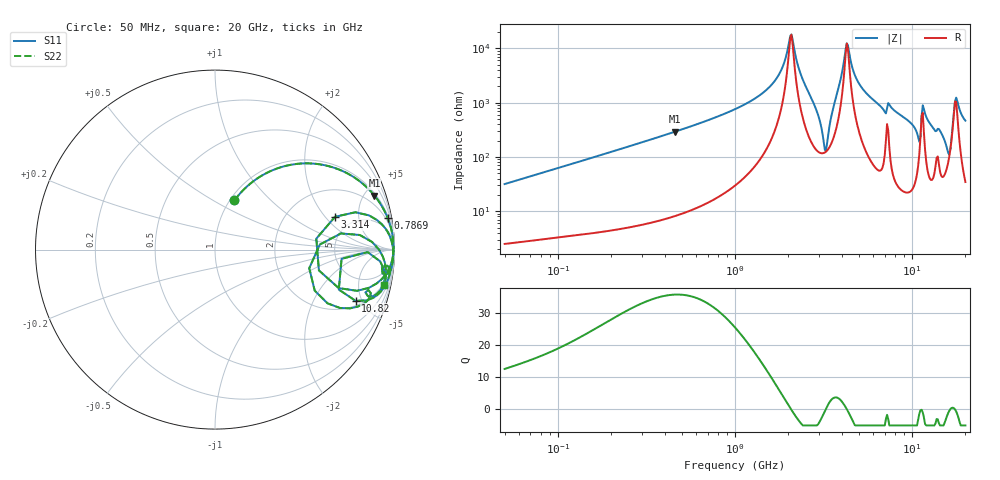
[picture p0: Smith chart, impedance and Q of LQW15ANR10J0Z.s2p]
!Murata Part Number: LQW15ANR10J0Z
!These Parameters are Measured in Series Mode Connection
!  o--[Z]--o
!Port1  Port2
!  o-------o
!Freq. Start=50[MHz] Stop=20[GHz], 401[Steps]
# Hz S RI R 50
!Freq.(Hz) S11(Real) S11(Imag) S21(Real) S21(Imag) S12(Real) S12(Imag) S22(Real) S22(Imag)
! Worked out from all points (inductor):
!   401 points, 50 MHz to 20 GHz, reference 50 ohm
!   read as one part in series: L = 99.7 nH near 51.52 MHz
!   highest Q = 35.8 at 458.9 MHz (marker M1), where L = 101 nH
!   self-resonance near 2.052 GHz
!   S11 on the Smith chart (normalised r, x): 50 MHz: 1.05, +0.63; 786.9 MHz: 1, +11; 3.314 GHz: 3.63, +2.56; 10.82 GHz: 2.37, -4.45; 20 GHz: 1.69, -9.30
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5e7  0.1085 0.274  0.8915 -0.274  0.8915 -0.274  0.1085 0.274
1.364002e8  0.4206 0.4722  0.5794 -0.4722  0.5794 -0.4722  0.4206 0.4722
3.721004e8  0.8382 0.3542  0.1618 -0.3542  0.1618 -0.3542  0.8382 0.3542
4.589149e8  0.8884 0.3013  0.1116 -0.3013  0.1116 -0.3013  0.8884 0.3013
7.868965e8  0.9621 0.1755  0.0379 -0.1755  0.0379 -0.1755  0.9621 0.1755
1e9  0.978 0.1283  0.022 -0.1283  0.022 -0.1283  0.978 0.1283
1.639343e9  0.9934 0.0429  0.00658 -0.0429  0.00658 -0.0429  0.9934 0.0429
2.083303e9  0.9945 -0.000765  0.00546 0.000765  0.00546 0.000765  0.9945 -0.000765
2.728004e9  0.9787 -0.0856  0.0213 0.0856  0.0213 0.0856  0.9787 -0.0856
3.121702e9  0.7913 -0.2296  0.2087 0.2296  0.2087 0.2296  0.7913 -0.2296
3.314454e9  0.6688 0.1828  0.3312 -0.1828  0.3312 -0.1828  0.6688 0.1828
3.572216e9  0.95 0.1169  0.05 -0.1169  0.05 -0.1169  0.95 0.1169
4.275624e9  0.992 0.000815  0.00798 -0.000815  0.00798 -0.000815  0.992 0.000815
5.273168e9  0.9914 -0.0554  0.00859 0.0554  0.00859 0.0554  0.9914 -0.0554
7.442007e9  0.9722 -0.1024  0.0278 0.1024  0.0278 0.1024  0.9722 -0.1024
1.082228e10  0.7835 -0.2855  0.2165 0.2855  0.2165 0.2855  0.7835 -0.2855
1.166392e10  0.9411 -0.11  0.0589 0.11  0.0589 0.11  0.9411 -0.11
1.460232e10  0.8481 -0.2858  0.1519 0.2858  0.1519 0.2858  0.8481 -0.2858
1.597544e10  0.5557 -0.229  0.4443 0.229  0.4443 0.229  0.5557 -0.229
1.670968e10  0.7019 0.0902  0.2981 -0.0902  0.2981 -0.0902  0.7019 0.0902
1.774144e10  0.9347 -0.0381  0.0653 0.0381  0.0653 0.0381  0.9347 -0.0381
2e10  0.9426 -0.1985  0.0574 0.1985  0.0574 0.1985  0.9426 -0.1985
